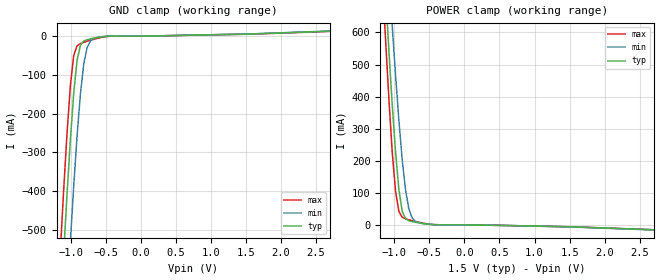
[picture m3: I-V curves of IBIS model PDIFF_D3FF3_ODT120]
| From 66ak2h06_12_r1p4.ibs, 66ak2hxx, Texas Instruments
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|   Model PDIFF_D3FF3_ODT120
[Model] PDIFF_D3FF3_ODT120
Model_type   Input
Polarity   Non-Inverting
Enable   Active-High
C_comp   3.275pF   3.214pF   3.363pF
C_comp_pullup   547.707fF   526.037fF   584.872fF
C_comp_pulldown 2.721pF   2.682pF   2.772pF
Vinh = 925.000mV
Vinl = 575.000mV
[Temperature Range]   25.000   125.000   -40.000
[Voltage Range]   1.500V   1.425V   1.575V
[GND Clamp Reference]   0.00V   0.00V   0.00V
|[C Comp Corner]
| variable   typ   min   max
|C_comp 3.275pF   3.363pF   3.214pF
|C_comp_pullup 547.707fF   584.872fF   526.037fF
|C_comp_pulldown 2.721pF   2.772pF   2.682pF
[POWER Clamp Reference]   1.500V   1.425V   1.575V
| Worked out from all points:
|   GND clamp passes 1 mA (typ) near -0.53 V on its own axis
|   POWER clamp passes 1 mA (typ) near -0.47 V on its own axis
[GND Clamp]
-1.48V    -1.914A    -2.176A    -1.76A
-1.145V   -720.2mA   -997.8mA   -553.4mA
-1.098V   -560.2mA   -836.7mA   -395.9mA
-1.05V    -407.4mA   -679.6mA   -249.9mA
-1.002V   -266.5mA   -528.6mA   -126.7mA
-954.6mV  -146.2mA   -386.2mA   -49.49mA
-906.8mV  -62.09mA   -257.1mA   -24.73mA
-859.1mV  -23.66mA   -148.8mA   -18.9mA
-811.4mV  -12.5mA    -71.27mA   -15.75mA
-715.9mV  -6.663mA   -12.09mA   -10.33mA
-572.7mV  -1.958mA   -1.649mA   -3.59mA
2.959V    14.61mA    15.11mA    14.05mA
[Power Clamp]
-1.459V   2.08A      2.199A     2.039A
-1.173V   907.9mA    1.125A     775.7mA
-1.125V   722.6mA    952.6mA    578.7mA
-1.077V   544mA      784.2mA    392.7mA
-1.03V    376mA      621.4mA    227.6mA
-981.8mV  226mA      466.6mA    104.3mA
-934.1mV  108.4mA    324.2mA    41.4mA
-886.4mV  41.57mA    201mA      23.36mA
-838.6mV  18.77mA    106.7mA    18.53mA
-790.9mV  12.51mA    48.2mA     15.51mA
-647.7mV  5.868mA    6.184mA    7.821mA
2.98V     -17.73mA   -18.39mA   -17.59mA
